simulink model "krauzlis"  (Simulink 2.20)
settings: Solver=ode45  StartTime=0.0  StopTime=2  MaxStep=.001  RelTol=1e-6  AbsTol=1e-6
libraries: simulink x2

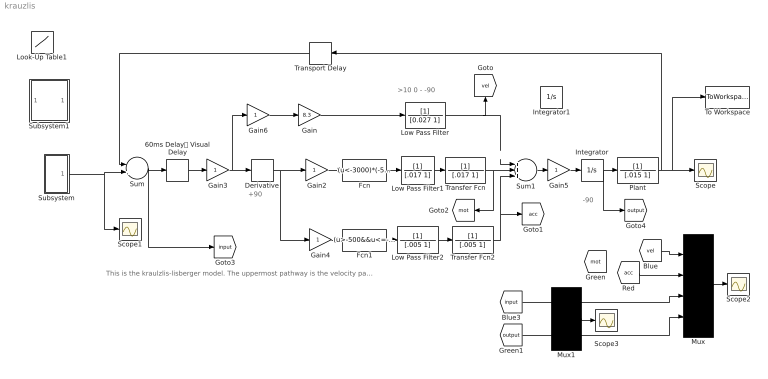
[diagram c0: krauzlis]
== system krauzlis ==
  note: 
  note: -90
  note: +90
  note: >10 0 - -90
  note: This is the kraulzlis-lisberger model. The uppermost pathway is the velocity pathway Next down is the initial acceleration pathway hich should give you the motion onset signal but seems broken in this implementation (Paul: fix it). The third pathway is the continuous velocity pathway. The most interesting thing to do is to consider the relative phase angles of the subcomponents and the effects of the terminal integrator. This integrator is private to pursuit (not the 'step' integrator which is bundled into the 'plant' box. Check this out by putting a set of scope inputs onto the three lines and viewing them before they are combined. The Intuition here is that the big difference between this model and the 'simplest' model in fig 6a is the terminal integrator whose 90 phase lag (with regard to the top/velocity line) is what is setting up the oscillations Note that to get the oscillations you need to get a 180 phase diff. In the notes stress how important it is to scope and compare the phase angles between signals at the beginning and end of the system. Think about which ones give you phase leads and lags and mention the bode plots for the functions and that below about 10Hz they dont contibute much to phase. The nest thing to be clear on is that the last integration doesnt actually screw up the top/velocity signal because initial eye accelleration is proportional to velocity There is a linear version of the model that works in a similar way but the non-linearities are really what allow you to match the data for early pursuit.
  60ms Delay Visual Delay : TransportDelay  DelayTime=.060  InitialInput=0  BufferSize=1024
  Derivative : Derivative
  Fcn : Fcn  Expr=(u<-3000)*(-5625*log(.00015*abs(u)+1))+(u>3000)*(5625*log(.00015*abs(u)+1))
  Fcn1 : Fcn  Expr=(u>-500&&u<=-25)*(-42*log(.1*abs(u)+1))+(u>-25&&u<=0)*(-(.0672*u^2)*log(.1*abs(u)+1))+(u>0&&u<=25)*((.0672*u^2)*log(.1*abs(u)+1))+(u>25&&u<=500)*(42*log(.1*abs(u)+1))
  Gain : Gain  Gain=8.3
  Gain{2..6} (5 alike) : Gain  Gain=1
  Integrator : Integrator  ExternalReset=none  InitialConditionSource=internal  InitialCondition=0  LimitOutput=off  UpperSaturationLimit=inf  LowerSaturationLimit=-inf  ShowSaturationPort=off  ShowStatePort=off  AbsoluteTolerance=auto
  Integrator1 : Integrator  ExternalReset=none  InitialConditionSource=internal  InitialCondition=0  LimitOutput=off  UpperSaturationLimit=inf  LowerSaturationLimit=-inf  ShowSaturationPort=off  ShowStatePort=off  AbsoluteTolerance=auto
  Look-Up Table1 : Lookup  InputValues=[-10000:10000]  OutputValues=[-5625*log(0.00015*(10000:-1:3001)+1) zeros(1,6001) 5625*log((3001:10000)*.00015+1)]
  Low Pass Filter : TransferFcn  Numerator=[1]  Denominator=[0.027 1]
  Low Pass Filter1 : TransferFcn  Numerator=[1]  Denominator=[.017 1]
  Low Pass Filter2 : TransferFcn  Numerator=[1]  Denominator=[.005 1]
  Mux : Mux  Inputs=4
  Mux1 : Mux  Inputs=2
  Plant : TransferFcn  Numerator=[1]  Denominator=[.015 1]
  Scope{,1..3} (4 alike) : Scope
  Subsystem : Subsystem
  Subsystem1 : Subsystem
  Sum : Sum  Inputs=-+
  Sum1 : Sum  Inputs=+++
  To Workspace : ToWorkspace  VariableName=simout  SampleTime=.01
  Transfer Fcn : TransferFcn  Numerator=[1]  Denominator=[.017 1]
  Transfer Fcn2 : TransferFcn  Numerator=[1]  Denominator=[.005 1]
  Transport Delay : TransportDelay  Orientation=left  DelayTime=0  InitialInput=0  BufferSize=1024
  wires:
  Transport Delay/1 -> Sum/1
  Gain/1 -> Low Pass Filter/1
  60ms Delay Visual Delay/1 -> Gain3/1
  Gain6/1 -> Gain/1
  Low Pass Filter1/1 -> Transfer Fcn/1
  Fcn/1 -> Low Pass Filter1/1
  Low Pass Filter2/1 -> Transfer Fcn2/1
  Fcn1/1 -> Low Pass Filter2/1
  Gain4/1 -> Fcn1/1
  Plant/1 -> Transport Delay/1, To Workspace/1, Scope/1
  Sum1/1 -> Gain5/1
  Gain3/1 -> Gain6/1, Derivative/1
  Gain5/1 -> Integrator/1
  Low Pass Filter/1 -> Sum1/1, [vel]
  Transfer Fcn2/1 -> Sum1/3, [acc]
  Transfer Fcn/1 -> Sum1/2, [mot]
  Mux/1 -> Scope2/1
  Subsystem/1(Out1) -> Sum/2, Scope1/1
  Derivative/1 -> Gain2/1, Gain4/1
  Sum/1 -> 60ms Delay Visual Delay/1, [input]
  Integrator/1 -> Plant/1, [output]
  [vel] -> Mux/1
  Mux1/1 -> Scope3/1
  Gain2/1 -> Fcn/1
  [acc] -> Mux/2
  [input] -> Mux/3
  [output] -> Mux/4

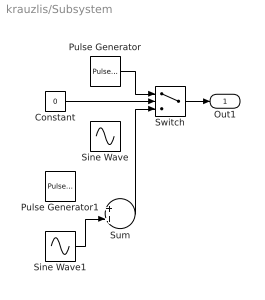
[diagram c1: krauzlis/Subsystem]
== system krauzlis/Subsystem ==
  Constant : Constant  Value=0
  Pulse Generator : simulink/Sources/Pulse Generator  period=100  duty=50  amplitude=20  start=0
  Pulse Generator1 : simulink/Sources/Pulse Generator  period=100  duty=50  amplitude=20  start=0
  Sine Wave : Sin  Amplitude=10  Frequency=10*pi*2  Phase=0  SampleTime=0
  Sine Wave1 : Sin  Amplitude=15  Frequency=1*pi*2  Phase=0  SampleTime=0
  Sum : Sum  Inputs=++
  Switch : Switch  Threshold=1
  Out1 : Outport  Port=1  InitialOutput=0
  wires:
  Pulse Generator/1 -> Switch/1
  Constant/1 -> Switch/2
  Switch/1 -> Out1/1
  Sine Wave1/1 -> Sum/2
  Sum/1 -> Switch/3

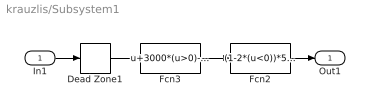
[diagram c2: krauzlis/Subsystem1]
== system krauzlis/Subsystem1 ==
  In1 : Inport  Port=1  PortWidth=-1  SampleTime=-1
  Dead Zone1 : DeadZone  LowerValue=-3000  UpperValue=3000
  Fcn2 : Fcn  Expr=(1-2*(u<0))*5625*log(.00015*abs(u)+1)
  Fcn3 : Fcn  Expr=u+3000*(u>0)-3000*(u<0)
  Out1 : Outport  Port=1  InitialOutput=0
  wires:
  Dead Zone1/1 -> Fcn3/1
  Fcn3/1 -> Fcn2/1
  In1/1 -> Dead Zone1/1
  Fcn2/1 -> Out1/1
